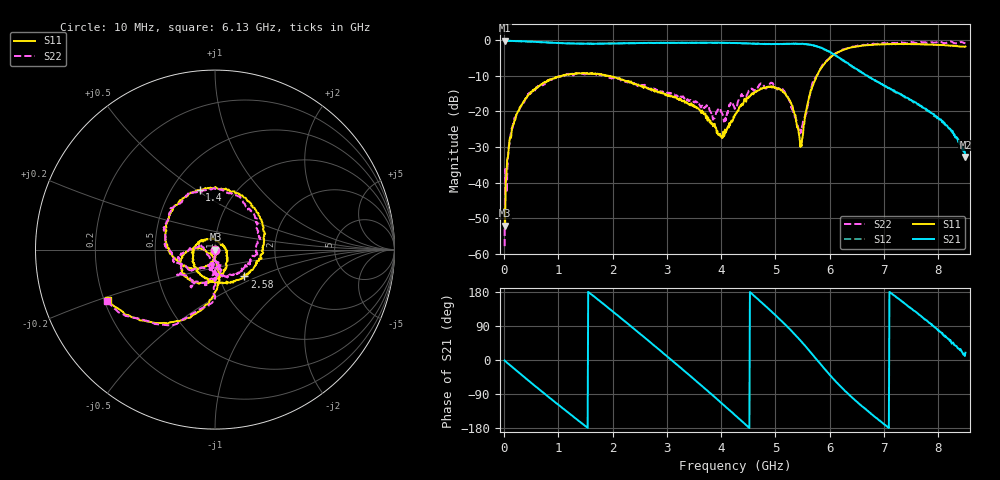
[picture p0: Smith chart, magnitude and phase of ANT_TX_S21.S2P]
!Agilent Technologies,E5071C,MY46523237,B.13.01
!Date: Tue Sep 12 16:53:57 2023
!Data & Calibration Information:
!Freq	S11:SOLT2(ON)	S21:SOLT2(ON)	S12:SOLT2(ON)	S22:SOLT2(ON)
!PortZ  Port1:50+j0  Port2:50+j0
!Above PortZ is port z conversion or system Z0 setting when saving the data.
!When reading, reference impedance value at option line is always used.
# Hz S dB R 50
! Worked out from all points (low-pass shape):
!   850 points, 10 MHz to 8.5 GHz, reference 50 ohm
!   highest |S21| = -0.08 dB at 20 MHz (marker M1); lowest = -32.8 dB at 8.5 GHz (marker M2)
!   |S21| within 3 dB of the highest: start of sweep to 5.977 GHz
!   lowest |S11| = -52.1 dB at 20 MHz (marker M3), VSWR 1.00, Z = 50.2 - j0.0311 ohm
!   |S11| at or under -10 dB: start of sweep to 1.067 GHz; 1.878754 GHz to 1.881423 GHz (2.669 MHz wide, 0.142 % of centre); 1.922 GHz to 5.764 GHz (3.842 GHz wide, 100 % of centre)
!   |S22| runs from -57.9 to -0.3 dB; largest |S21 - S12| = 0.013
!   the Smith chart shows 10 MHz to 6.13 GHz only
!   S11 on the Smith chart (normalised r, x): 10 MHz: 1.00, -0.01; 1.4 GHz: 0.69, +0.52; 2.58 GHz: 1.32, -0.41; 6.13 GHz: 0.21, -0.21
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1e7  -47.47 -96.0  -0.08 -1.3  -0.05 -1.5  -57.86 -85.8
2e7  -52.10 -7.2  -0.08 -2.8  -0.12 -2.9  -36.18 6.3
1.1e8  -27.31 -86.8  -0.18 -13.6  -0.16 -13.6  -27.61 -96.7
2.8e8  -19.37 -118.6  -0.25 -33.9  -0.26 -34.0  -19.55 -113.9
7.9e8  -11.45 177.1  -0.59 -94.2  -0.62 -94.0  -11.39 178.4
1.4e9  -9.30 104.4  -0.96 -163.3  -0.93 -163.5  -9.32 113.6
1.43e9  -9.29 101.3  -0.94 -166.6  -0.95 -166.8  -9.35 110.1
2.09e9  -10.74 22.4  -0.89 118.3  -0.87 118.0  -10.73 40.6
2.58e9  -13.11 -42.5  -0.72 60.0  -0.77 60.2  -12.62 -6.3
2.84e9  -14.70 -81.3  -0.72 29.2  -0.72 29.3  -14.46 -27.5
3.66e9  -20.35 157.9  -0.70 -70.2  -0.71 -70.4  -18.97 -99.8
4.26e9  -21.02 -41.3  -0.80 -146.0  -0.79 -146.3  -18.85 -81.9
4.66e9  -14.22 -106.5  -0.96 162.6  -0.96 162.4  -13.81 -119.8
5.1e9  -14.08 -163.6  -1.02 104.7  -1.06 104.3  -13.67 -167.9
5.47e9  -28.89 -124.0  -1.03 49.8  -0.99 49.9  -25.07 -121.5
5.67e9  -13.52 -86.5  -1.40 16.6  -1.35 17.2  -12.74 -91.5
6.13e9  -3.60 -154.9  -4.42 -59.9  -4.51 -59.4  -3.52 -154.4
6.56e9  -1.64 147.3  -8.76 -117.4  -8.75 -117.2  -1.46 151.0
7.09e9  -1.07 82.0  -13.35 -179.6  -13.44 -178.8  -0.69 96.5
7.8e9  -1.23 -9.9  -19.57 102.5  -19.91 101.3  -0.74 31.2
8.19e9  -1.45 -70.1  -24.68 55.2  -24.39 53.8  -0.54 -7.3
8.5e9  -1.77 -128.2  -32.79 19.2  -32.43 12.3  -0.84 -37.7
